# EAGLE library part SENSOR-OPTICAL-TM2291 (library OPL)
Infrared sensor signal processor
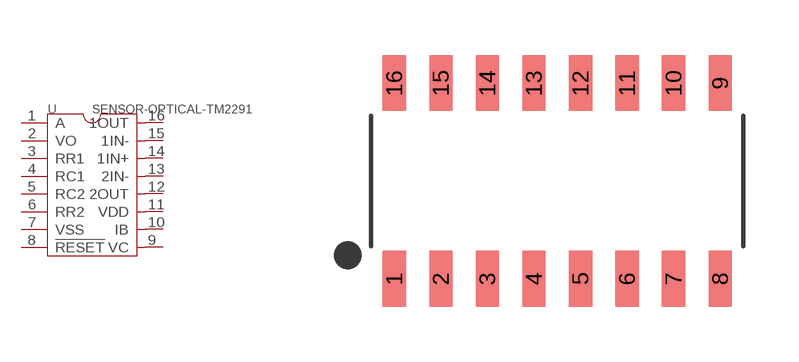
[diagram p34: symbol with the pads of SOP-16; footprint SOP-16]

Designator prefix U

## SENSOR-OPTICAL-TM2291-314020020  [SOP-16]
1  A
2  VO
3  RR1
4  RC1
5  RC2
6  RR2
7  VSS  sup
8  !RESET  in
9  VC
10  IB
11  VDD  sup
12  2OUT  out
13  2IN-  in
14  1IN+  in
15  1IN-  in
16  1OUT  out

## Footprint SOP-16 (pad centres in mm)
smd 0.635 x 1.524: 1 -4.445,-2.667; 2 -3.175,-2.667; 3 -1.905,-2.667; 4 -0.635,-2.667; 5 0.635,-2.667; 6 1.905,-2.667; 7 3.175,-2.667; 8 4.445,-2.667; 9 4.445,2.667; 10 3.175,2.667; 11 1.905,2.667; 12 0.635,2.667; 13 -0.635,2.667; 14 -1.905,2.667; 15 -3.175,2.667; 16 -4.445,2.667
